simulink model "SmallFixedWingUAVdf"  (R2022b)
settings: Solver=ode4  StartTime=0  StopTime=stoptime  FixedStep=0.001  RelTol=1e-3  EnableMultiTasking=on
PreLoadFcn:
  | asbswarm_vehicledata; % load in workspace variables
PostLoadFcn:
  | open_system([gcs,'/MATLAB Animation Display/MATLAB',10,'Animation']);
InitFcn:
  | InitDatactrl
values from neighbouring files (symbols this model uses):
  env = struct    [InitDatactrl.m]
  F = Fattr + Frep    [APF.m]
  q = ix-1    [bspline_deboor.m]
  SenorSampleTime = 0.01    [InitDatactrl.m]
  sensors = struct    [InitDatactrl.m]
  uav = struct    [InitDatactrl.m]    (also in InitDatactrldf.m)
undefined symbols (not defined in the file or in its folder): Busy, Continuous, DiscIntNeverNeededParam, Dryden, Earth, Light, MIL, Newton, pa28, r, Raphson, sigbuilder_block, Wait, WGS84
libraries: simulink x37, aerolibactuator x10, sharedtransform x6, aerolibatmos2 x4, aerolibasang x4, aerolibwind2 x4, aerolibtransform2 x3, aerolibconvert2 x3, aerolibfltsims x2, shared6dof x2, aerolibnav x2, aerolibanimutils x1
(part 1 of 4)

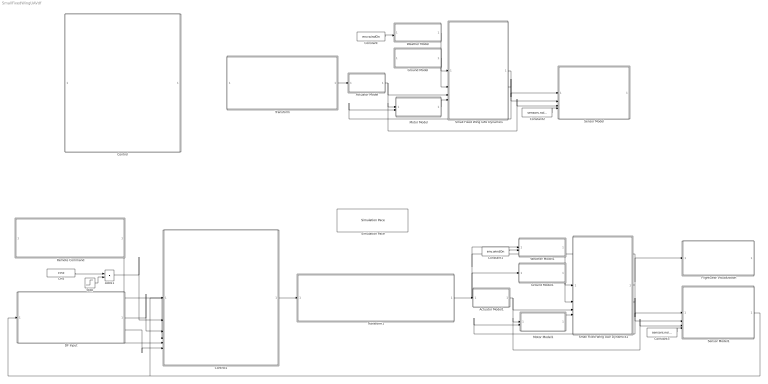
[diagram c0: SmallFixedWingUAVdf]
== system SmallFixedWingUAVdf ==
  Actuator Model : Subsystem  Commented=on
  Actuator Model1 : Subsystem
  Add11 : Sum
  CH5 : Constant  Value=1550  OutDataTypeStr=single
  Constant : Constant  Commented=on  Value=env.windOn
  Constant1 : Constant  Value=env.windOn
  Constant2 : Constant  Commented=on  Value=sensors.noiseOn
  Constant3 : Constant  Value=sensors.noiseOn
  Control : Subsystem  Commented=on
  Control1 : Subsystem
  DF Input : Subsystem
  FlightGear Visualization : Subsystem
  Ground Model : Subsystem  Commented=on
  Ground Model1 : Subsystem
  Motor Model : Subsystem  Commented=on
  Motor Model1 : Subsystem
  Remote Command : Subsystem
  Sensor Model : Subsystem  Commented=on
  Sensor Model1 : Subsystem
  Simulation Pace : aerolibanimutils/Simulation Pace  SimulationPace=1  SleepMode=Busy-Wait  OutputPaceError=off  SampleTime=-1
  Small Fixed Wing UAV Dynamics : Subsystem  Commented=on
  Small Fixed Wing UAV Dynamics1 : Subsystem
  Step : Step  Time=0  After=-100  SampleTime=0
  Transform : Subsystem  Commented=on
  Transform1 : Subsystem
  Weather Model : Subsystem  Commented=on
  Weather Model1 : Subsystem
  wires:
  Small Fixed Wing UAV Dynamics/1(UAVState) -> Sensor Model/1(UAVState)
  Step/1 -> Add11/2
  Motor Model/1(Motor F_M) -> Small Fixed Wing UAV Dynamics/4(Motor Thrust)
  Small Fixed Wing UAV Dynamics/2(AirData) -> Motor Model/2(Air Data), Sensor Model/2(AirData)
  Transform/1(Actuator_act) -> Actuator Model/1(CtrlCmds)
  Actuator Model/1(CtrlSurfaces) -> Small Fixed Wing UAV Dynamics/3(CtrlSurfaces), Sensor Model/3(CtrlSurfaces), Motor Model/1(Ctrl Surfaces)
  Constant2/1 -> Sensor Model/4(if Noise)
  Weather Model/1(Wind_e) -> Small Fixed Wing UAV Dynamics/1(Wind_e)
  Constant/1 -> Weather Model/2(if Wind On)
  CH5/1 -> Add11/1
  Ground Model/1(if Ground) -> Small Fixed Wing UAV Dynamics/2(Ground Detection)
  Actuator Model1/1(CtrlSurfaces) -> Small Fixed Wing UAV Dynamics1/3(CtrlSurfaces), Sensor Model1/3(CtrlSurfaces), Motor Model1/1(Ctrl Surfaces)
  Transform1/1(Actuator_act) -> Actuator Model1/1(CtrlCmds)
  Small Fixed Wing UAV Dynamics1/2(AirData) -> Motor Model1/2(Air Data), Sensor Model1/2(AirData)
  Control1/1(Actuator) -> Transform1/1(Actuator_cmd)
  Constant3/1 -> Sensor Model1/4(if Noise)
  Motor Model1/1(Motor F_M) -> Small Fixed Wing UAV Dynamics1/4(Motor Thrust)
  Ground Model1/1(if Ground) -> Small Fixed Wing UAV Dynamics1/2(Ground Detection)
  Constant1/1 -> Weather Model1/2(if Wind On)
  Weather Model1/1(Wind_e) -> Small Fixed Wing UAV Dynamics1/1(Wind_e)
  Small Fixed Wing UAV Dynamics1/1(UAVState) -> FlightGear Visualization/1(UAVState), Weather Model1/1(UavState), Ground Model1/1(UavState), Sensor Model1/1(UAVState)
  Remote Command/1(Command) -> Control1/1(Command)
  Add11/1 -> Control1/2(ch_switch)
  DF Input/1(RollCmd_Nav) -> Control1/3(RollCmd)
  DF Input/2(AltitudeCmd_Nav) -> Control1/5(AltitudeCmd)
  DF Input/3(AccCmd_Nav) -> Control1/7(AccCmd)
  Sensor Model1/1(SensorData) -> DF Input/1(SensorData), Control1/4(SensorData)

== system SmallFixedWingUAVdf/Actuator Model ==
  note: Simple Actuator Model
  CtrlCmds : Inport
  Bus Creator1 : BusCreator  Inputs=5
  Bus Selector : BusSelector  OutputSignals=elevatorCmd,aileronCmd,rudderCmd,flapCmd,throttleCmd
  Data Type Conversion{1..4,7} (5 alike) : DataTypeConversion  OutDataTypeStr=double
  Linear Second Order Actuators : aerolibactuator/Linear Second-Order Actuator  wn_fin=35  z_fin=0.75  fin_act_0=0  fin_act_vel=0
  Linear Second-Order Actuator{1..4} (4 alike) : aerolibactuator/Linear Second-Order Actuator  wn_fin=35  z_fin=0.75  fin_act_0=0  fin_act_vel=0
  Signal Specification{,1..3} (4 alike) : SignalSpecification  Unit=rad
  Signal Specification4 : SignalSpecification  Unit=%
  CtrlSurfaces : Outport  VectorParamsAs1DForOutWhenUnconnected=off
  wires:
  CtrlCmds/1 -> Bus Selector/1
  Data Type Conversion7/1 -> Linear Second-Order Actuator4/1
  Data Type Conversion1/1 -> Linear Second-Order Actuator3/1
  Data Type Conversion2/1 -> Linear Second-Order Actuator2/1
  Data Type Conversion3/1 -> Linear Second-Order Actuator1/1
  Data Type Conversion4/1 -> Linear Second Order Actuators/1
  Bus Creator1/1 -> CtrlSurfaces/1
  Bus Selector/1 -> Data Type Conversion7/1  "<elevatorCmd>"
  Linear Second-Order Actuator2/1 -> Signal Specification2/1
  Linear Second-Order Actuator3/1 -> Signal Specification1/1
  Linear Second-Order Actuator1/1 -> Signal Specification3/1
  Linear Second-Order Actuator4/1 -> Signal Specification/1
  Bus Selector/4 -> Data Type Conversion3/1  "<flapCmd>"
  Bus Selector/5 -> Data Type Conversion4/1  "<throttleCmd>"
  Bus Selector/3 -> Data Type Conversion2/1  "<rudderCmd>"
  Bus Selector/2 -> Data Type Conversion1/1  "<aileronCmd>"
  Linear Second Order Actuators/1 -> Signal Specification4/1
  Signal Specification/1 -> Bus Creator1/1  "dE"
  Signal Specification1/1 -> Bus Creator1/2  "dA"
  Signal Specification2/1 -> Bus Creator1/3  "dR"
  Signal Specification3/1 -> Bus Creator1/4  "dF"
  Signal Specification4/1 -> Bus Creator1/5  "dT"

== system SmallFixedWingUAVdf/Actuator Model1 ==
  note: Simple Actuator Model
  CtrlCmds : Inport
  Bus Creator1 : BusCreator  Inputs=5
  Bus Selector : BusSelector  OutputSignals=elevatorCmd,aileronCmd,rudderCmd,flapCmd,throttleCmd
  Data Type Conversion{1..4,7} (5 alike) : DataTypeConversion  OutDataTypeStr=double
  Linear Second Order Actuators : aerolibactuator/Linear Second-Order Actuator  wn_fin=35  z_fin=0.75  fin_act_0=0  fin_act_vel=0
  Linear Second-Order Actuator{1..4} (4 alike) : aerolibactuator/Linear Second-Order Actuator  wn_fin=35  z_fin=0.75  fin_act_0=0  fin_act_vel=0
  Signal Specification{,1..3} (4 alike) : SignalSpecification  Unit=rad
  Signal Specification4 : SignalSpecification  Unit=%
  CtrlSurfaces : Outport  VectorParamsAs1DForOutWhenUnconnected=off
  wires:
  CtrlCmds/1 -> Bus Selector/1
  Data Type Conversion7/1 -> Linear Second-Order Actuator4/1
  Data Type Conversion1/1 -> Linear Second-Order Actuator3/1
  Data Type Conversion2/1 -> Linear Second-Order Actuator2/1
  Data Type Conversion3/1 -> Linear Second-Order Actuator1/1
  Data Type Conversion4/1 -> Linear Second Order Actuators/1
  Bus Creator1/1 -> CtrlSurfaces/1
  Bus Selector/1 -> Data Type Conversion7/1  "<elevatorCmd>"
  Linear Second-Order Actuator2/1 -> Signal Specification2/1
  Linear Second-Order Actuator3/1 -> Signal Specification1/1
  Linear Second-Order Actuator1/1 -> Signal Specification3/1
  Linear Second-Order Actuator4/1 -> Signal Specification/1
  Bus Selector/4 -> Data Type Conversion3/1  "<flapCmd>"
  Bus Selector/5 -> Data Type Conversion4/1  "<throttleCmd>"
  Bus Selector/3 -> Data Type Conversion2/1  "<rudderCmd>"
  Bus Selector/2 -> Data Type Conversion1/1  "<aileronCmd>"
  Linear Second Order Actuators/1 -> Signal Specification4/1
  Signal Specification/1 -> Bus Creator1/1  "dE"
  Signal Specification1/1 -> Bus Creator1/2  "dA"
  Signal Specification2/1 -> Bus Creator1/3  "dR"
  Signal Specification3/1 -> Bus Creator1/4  "dF"
  Signal Specification4/1 -> Bus Creator1/5  "dT"

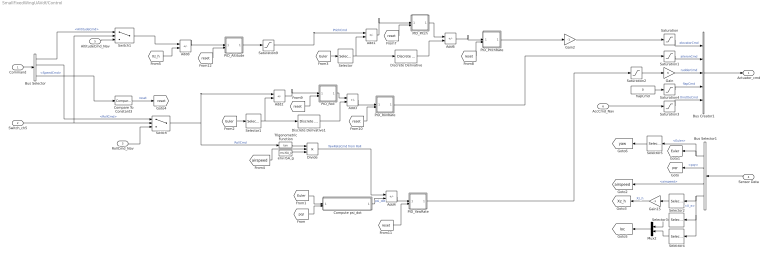
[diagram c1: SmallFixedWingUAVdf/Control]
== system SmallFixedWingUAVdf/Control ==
  Command : Inport
  Switch_ch5 : Inport  Port=2
  RollCmd_Nav : Inport  Port=3
  Sensor Data : Inport  Port=4
  AltitudeCmd_Nav : Inport  Port=5
  AccCmd_Nav : Inport  Port=6
  Add{1..4,6,8} (6 alike) : Sum  Inputs=+-
  Bus Creator1 : BusCreator  Inputs=5
  Bus Selector : BusSelector  OutputSignals=AlititudeCmd,RollCmd,YawRateCmd,SpeedCmd
  Bus Selector1 : BusSelector  OutputSignals=Euler,pqr,airspeed,X_e
  Compare To Constant3 : simulink/Logic and Bit Operations/Compare To Constant  relop=<=  const=0.1  OutDataTypeStr=boolean
  Compute psi_dot : Subsystem
  Discrete Derivative : simulink/Discrete/Discrete Derivative  gainval=1.0  ICPrevScaledInput=0.0  OutMin=[]  OutMax=[]  OutDataType=fixdt(1, 16)  OutScaling=2^-10  DoSatur=off
  Discrete Derivative1 : simulink/Discrete/Discrete Derivative  gainval=1.0  ICPrevScaledInput=0.0  OutMin=[]  OutMax=[]  OutDataType=fixdt(1, 16)  OutScaling=2^-10  DoSatur=off
  Divide : Product  Inputs=*/*
  Gain : Gain
  Gain15 : Gain  Gain=-1
  Gain2 : Gain  Gain=-1
  Mux2 : Mux  Inputs=2
  PID_Altitude : Subsystem
  PID_Pitch : Subsystem
  PID_PitchRate : Subsystem
  PID_Roll : Subsystem
  PID_RollRate : Subsystem
  PID_YawRate : Subsystem
  Saturation : Saturate  UpperLimit=uav.elevator.max  LowerLimit=uav.elevator.min
  Saturation1 : Saturate  UpperLimit=uav.aileron.max  LowerLimit=uav.aileron.min
  Saturation2 : Saturate  UpperLimit=uav.rudder.max  LowerLimit=uav.rudder.min
  Saturation3 : Saturate  UpperLimit=uav.throttlepercent.max  LowerLimit=uav.throttlepercent.min
  Saturation4 : Saturate  UpperLimit=uav.flap.max  LowerLimit=uav.flap.min
  Saturation9 : Saturate  UpperLimit=uav.attitudectrlmax.pitch  LowerLimit=-uav.attitudectrlmax.pitch
  Selector : Selector  InputPortWidth=3  IndexOptions=Index vector (dialog)  Indices=2  OutputSizes=1
  Selector1 : Selector  InputPortWidth=3  IndexOptions=Index vector (dialog)  Indices=1  OutputSizes=1
  Selector2 : Selector  InputPortWidth=3  IndexOptions=Index vector (dialog)  Indices=3  OutputSizes=1
  Selector3 : Selector  InputPortWidth=3  IndexOptions=Index vector (dialog)  Indices=1  OutputSizes=1
  Selector4 : Selector  InputPortWidth=3  IndexOptions=Index vector (dialog)  Indices=2  OutputSizes=1
  Selector5 : Selector  InputPortWidth=3  IndexOptions=Index vector (dialog)  Indices=3  OutputSizes=1
  Switch : Switch  Criteria=u2 > Threshold  Threshold=1500
  Switch1 : Switch  Criteria=u2 > Threshold  Threshold=1500
  Trigonometric Function : Trigonometry  Operator=tan
  env.ISA_g : Constant  Value=env.ISA_g
  flapCmd : Constant  Value=0  OutDataTypeStr=double
  Actuator_cmd : Outport
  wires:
  Saturation1/1 -> Bus Creator1/2  "aileronCmd"
  Add1/1 -> PID_Pitch/1(x)
  Selector3/1 -> Mux2/1
  Bus Selector1/4 -> Selector3/1, Selector4/1, Selector2/1  "<X_e>"
  PID_PitchRate/1(y) -> Gain2/1
  Bus Selector1/1 -> Selector5/1, [Euler]  "<Euler>"
  PID_Altitude/1(y) -> Saturation9/1
  RollCmd_Nav/1 -> Switch/3
  Saturation9/1 -> Add1/1  "PtichCmd"
  Add8/1 -> PID_Altitude/1(x)
  Gain15/1 -> [Xz_h]  "Xz_h"
  [pqr] -> Compute psi_dot/2(G)
  Gain/1 -> Bus Creator1/3  "rudderCmd"
  Selector/1 -> Discrete Derivative/1, Add1/2
  [Xz_h] -> Add8/2
  flapCmd/1 -> Saturation4/1
  [reset] -> PID_Pitch/2(reset_i)
  Bus Selector/2 -> Switch/1  "<RollCmd>"
  Compute psi_dot/1(psi_dot) -> Add4/2  "psi_dot"
  Add6/1 -> PID_PitchRate/1(x)
  Selector2/1 -> Gain15/1
  Bus Selector1/2 -> [pqr]  "<pqr>"
  Selector4/1 -> Mux2/2
  [Euler] -> Compute psi_dot/1(Euler)
  Saturation3/1 -> Bus Creator1/5  "throttleCmd"
  [Euler] -> Selector/1
  Sensor Data/1 -> Bus Selector1/1
  env.ISA_g/1 -> Divide/3
  Add4/1 -> PID_YawRate/1(x)
  [airspeed] -> Divide/2
  Switch/1 -> Add2/1, Trigonometric Function/1  "RollCmd"
  Saturation4/1 -> Bus Creator1/4  "flapCmd"
  Saturation/1 -> Bus Creator1/1  "elevatorCmd"
  PID_Pitch/1(y) -> Add6/1
  Saturation2/1 -> Gain/1
  Discrete Derivative/1 -> Add6/2
  Gain2/1 -> Saturation/1
  Bus Selector/4 -> Compare To Constant3/1  "<SpeedCmd>"
  Divide/1 -> Add4/1  "YawRateCmd from Roll"
  [reset] -> PID_Altitude/2(reset_i)
  PID_YawRate/1(y) -> Saturation2/1
  [reset] -> PID_YawRate/2(reset_i)
  [reset] -> PID_PitchRate/2(reset_i)
  Trigonometric Function/1 -> Divide/1
  Bus Selector1/3 -> [airspeed]  "<airspeed>"
  Command/1 -> Bus Selector/1
  Switch_ch5/1 -> Switch/2, Switch1/2
  Bus Creator1/1 -> Actuator_cmd/1
  Compare To Constant3/1 -> [reset]  "reset"
  Mux2/1 -> [loc]
  Selector5/1 -> [yaw]
  Bus Selector/1 -> Switch1/1  "<AlititudeCmd>"
  Switch1/1 -> Add8/1
  AltitudeCmd_Nav/1 -> Switch1/3
  AccCmd_Nav/1 -> Saturation3/1
  Add2/1 -> PID_Roll/1(x)
  Discrete Derivative1/1 -> Add3/2
  [Euler] -> Selector1/1
  [reset] -> PID_Roll/2(reset_i)
  Selector1/1 -> Discrete Derivative1/1, Add2/2
  PID_Roll/1(y) -> Add3/1
  [reset] -> PID_RollRate/2(reset_i)
  Add3/1 -> PID_RollRate/1(x)
  PID_RollRate/1(y) -> Saturation1/1

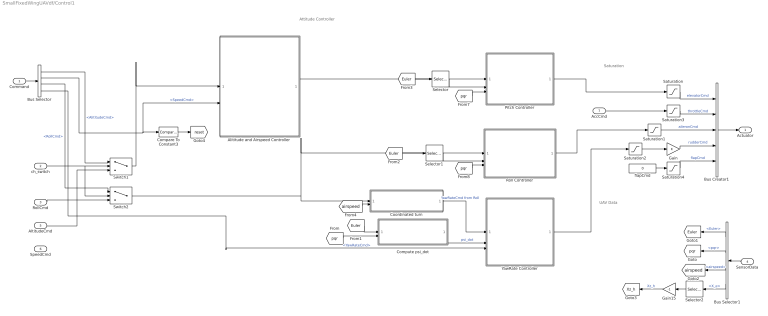
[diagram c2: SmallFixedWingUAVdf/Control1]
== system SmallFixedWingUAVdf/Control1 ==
  note: Attitude Controller
  note: UAV Data
  note: Saturation
  Command : Inport
  ch_switch : Inport  Port=2
  RollCmd : Inport  Port=3
  SensorData : Inport  Port=4
  AltitudeCmd : Inport  Port=5
  SpeedCmd : Inport  Port=6
  AccCmd : Inport  Port=7
  Alititude and Airspeed Controller : Subsystem
  Bus Creator1 : BusCreator  Inputs=5
  Bus Selector : BusSelector  OutputSignals=AlititudeCmd,SpeedCmd,RollCmd,YawRateCmd
  Bus Selector1 : BusSelector  OutputSignals=Euler,pqr,airspeed,X_e
  Compare To Constant3 : simulink/Logic and Bit Operations/Compare To Constant  relop=<=  const=0.2  OutDataTypeStr=boolean
  Compute psi_dot : Subsystem
  Coordinated turn : Subsystem
  Gain : Gain
  Gain15 : Gain  Gain=-1
  Pitch Controller : Subsystem
  Roll Controller : Subsystem
  Saturation : Saturate  UpperLimit=uav.elevator.max  LowerLimit=uav.elevator.min
  Saturation1 : Saturate  UpperLimit=uav.aileron.max  LowerLimit=uav.aileron.min
  Saturation2 : Saturate  UpperLimit=uav.rudder.max  LowerLimit=uav.rudder.min
  Saturation3 : Saturate  UpperLimit=uav.throttlepercent.max  LowerLimit=uav.throttlepercent.min
  Saturation4 : Saturate  UpperLimit=uav.flap.max  LowerLimit=uav.flap.min
  Selector : Selector  InputPortWidth=3  IndexOptions=Index vector (dialog)  Indices=2  OutputSizes=1
  Selector1 : Selector  InputPortWidth=3  IndexOptions=Index vector (dialog)  Indices=1  OutputSizes=1
  Selector2 : Selector  InputPortWidth=3  IndexOptions=Index vector (dialog)  Indices=3  OutputSizes=1
  Switch1 : Switch  Criteria=u2 > Threshold  Threshold=1500
  Switch2 : Switch  Criteria=u2 > Threshold  Threshold=1500
  YawRate Controller : Subsystem
  flapCmd : Constant  Value=0  OutDataTypeStr=double
  Actuator : Outport
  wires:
  Bus Selector1/3 -> [airspeed]  "<airspeed>"
  Pitch Controller/1(elevatorCmd) -> Saturation/1
  [airspeed] -> Coordinated turn/2(<airpseed>)
  [pqr] -> Roll Controller/3(pqr)
  [pqr] -> Pitch Controller/3(pqr)
  Saturation4/1 -> Bus Creator1/5  "flapCmd"
  [Euler] -> Compute psi_dot/1(Euler)
  Bus Selector/1 -> Switch1/1  "<AlititudeCmd>"
  Saturation/1 -> Bus Creator1/1  "elevatorCmd"
  Selector/1 -> Pitch Controller/2(Pitch act)
  Selector1/1 -> Roll Controller/2(Roll act)
  SensorData/1 -> Bus Selector1/1
  Bus Selector1/4 -> Selector2/1  "<X_e>"
  Saturation3/1 -> Bus Creator1/2  "throttleCmd"
  Compare To Constant3/1 -> [reset]
  YawRate Controller/1(rudderCmd) -> Saturation2/1
  Roll Controller/1(aileronCmd) -> Saturation1/1
  Bus Selector1/2 -> [pqr]  "<pqr>"
  [pqr] -> Compute psi_dot/2(G)
  flapCmd/1 -> Saturation4/1
  Selector2/1 -> Gain15/1
  Command/1 -> Bus Selector/1
  Bus Selector/4 -> YawRate Controller/3(<YawRateCmd>)  "<YawRateCmd>"
  [Euler] -> Selector1/1
  Saturation1/1 -> Bus Creator1/3  "aileronCmd"
  Bus Selector1/1 -> [Euler]  "<Euler>"
  Bus Selector/2 -> Alititude and Airspeed Controller/2(<SpeedCmd>), Compare To Constant3/1  "<SpeedCmd>"
  Bus Creator1/1 -> Actuator/1
  Gain/1 -> Bus Creator1/4  "rudderCmd"
  [Euler] -> Selector/1
  Compute psi_dot/1(psi_dot) -> YawRate Controller/2(psi_dot)  "psi_dot"
  Gain15/1 -> [Xz_h]  "Xz_h"
  Coordinated turn/1(YawRateCmd) -> YawRate Controller/1(psi_dot Cmd)  "YawRateCmd from Roll"
  Bus Selector/3 -> Switch2/1  "<RollCmd>"
  Saturation2/1 -> Gain/1
  Alititude and Airspeed Controller/1(pitchout) -> Pitch Controller/1(Pitch cmd)
  ch_switch/1 -> Switch2/2, Switch1/2
  AltitudeCmd/1 -> Switch1/3
  RollCmd/1 -> Switch2/3
  Switch1/1 -> Alititude and Airspeed Controller/1(<AlititudeCmd>)
  AccCmd/1 -> Saturation3/1
  Switch2/1 -> Coordinated turn/1(<RollCmd>), Roll Controller/1(Roll cmd)

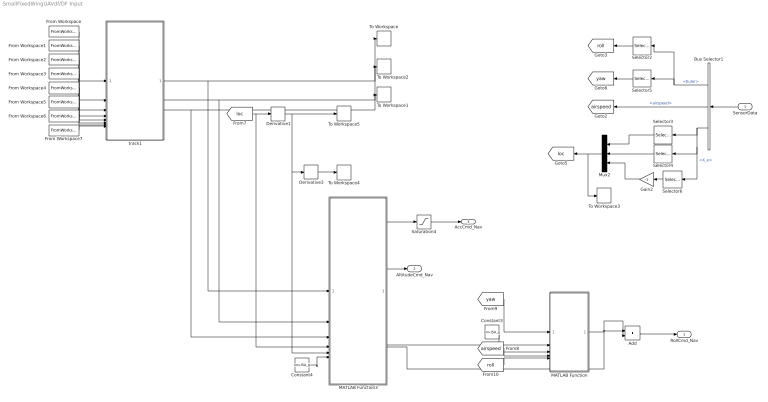
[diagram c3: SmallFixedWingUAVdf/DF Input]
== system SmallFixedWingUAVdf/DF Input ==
  SensorData : Inport
  Add : Sum
  Bus Selector1 : BusSelector  OutputSignals=Euler,airspeed,X_e
  Constant3 : Constant  Value=env.ISA_g
  Constant4 : Constant  Value=env.ISA_g
  Derivative1 : Derivative
  Derivative3 : Derivative
  From Workspace : FromWorkspace  VariableName=xts  SampleTime=-1
  From Workspace1 : FromWorkspace  VariableName=yts  SampleTime=-1
  From Workspace2 : FromWorkspace  VariableName=dxts  SampleTime=-1
  From Workspace3 : FromWorkspace  VariableName=dyts  SampleTime=-1
  From Workspace4 : FromWorkspace  VariableName=ddxts  SampleTime=-1
  From Workspace5 : FromWorkspace  VariableName=ddyts  SampleTime=-1
  From Workspace6 : FromWorkspace  VariableName=dddxts  SampleTime=-1
  From Workspace7 : FromWorkspace  VariableName=dddyts  SampleTime=-1
  Gain2 : Gain  Gain=-1
  MATLAB Function : MATLAB Function  TreatAsAtomicUnit=on
  MATLAB Function3 : MATLAB Function  TreatAsAtomicUnit=on
  Mux2 : Mux  Inputs=3
  Saturation4 : Saturate  UpperLimit=30  LowerLimit=-30
  Selector2 : Selector  InputPortWidth=3  IndexOptions=Index vector (dialog)  Indices=1  OutputSizes=1
  Selector3 : Selector  InputPortWidth=3  IndexOptions=Index vector (dialog)  Indices=1  OutputSizes=1
  Selector4 : Selector  InputPortWidth=3  IndexOptions=Index vector (dialog)  Indices=2  OutputSizes=1
  Selector5 : Selector  InputPortWidth=3  IndexOptions=Index vector (dialog)  Indices=3  OutputSizes=1
  Selector6 : Selector  InputPortWidth=3  IndexOptions=Index vector (dialog)  Indices=3  OutputSizes=1
  To Workspace : ToWorkspace  VariableName=Xd  SampleTime=0.1
  To Workspace1 : ToWorkspace  VariableName=Ad  SampleTime=0.1
  To Workspace2 : ToWorkspace  VariableName=Vd  SampleTime=0.1
  To Workspace3 : ToWorkspace  VariableName=X  SampleTime=0.1
  To Workspace4 : ToWorkspace  VariableName=A  SampleTime=0.1
  To Workspace5 : ToWorkspace  VariableName=V  SampleTime=0.1
  track1 : MATLAB Function  TreatAsAtomicUnit=on
  RollCmd_Nav : Outport
  AltitudeCmd_Nav : Outport  Port=2
  AccCmd_Nav : Outport  Port=3
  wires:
  Bus Selector1/3 -> Selector6/1, Selector4/1, Selector3/1  "<X_e>"
  Selector4/1 -> Mux2/2
  Mux2/1 -> [loc], To Workspace3/1
  Bus Selector1/2 -> [airspeed]  "<airspeed>"
  Selector3/1 -> Mux2/1
  Bus Selector1/1 -> Selector2/1, Selector5/1  "<Euler>"
  Selector5/1 -> [yaw]
  SensorData/1 -> Bus Selector1/1
  From Workspace3/1 -> track1/4(dy)
  From Workspace6/1 -> track1/7(dddx)
  From Workspace7/1 -> track1/8(dddy)
  From Workspace1/1 -> track1/2(y)
  track1/2(Vd) -> MATLAB Function3/2(dxd), To Workspace2/1
  From Workspace2/1 -> track1/3(dx)
  track1/1(Xd) -> MATLAB Function3/1(xd), To Workspace/1
  Derivative3/1 -> To Workspace4/1
  From Workspace5/1 -> track1/6(ddy)
  From Workspace4/1 -> track1/5(ddx)
  track1/3(Ad) -> MATLAB Function3/3(ddxd), To Workspace1/1
  From Workspace/1 -> track1/1(x)
  Selector2/1 -> [roll]
  [loc] -> MATLAB Function3/4(x), Derivative1/1
  Selector6/1 -> Gain2/1
  Gain2/1 -> Mux2/3
  Derivative1/1 -> MATLAB Function3/5(dx), Derivative3/1, To Workspace5/1
  MATLAB Function3/2(Hz) -> AltitudeCmd_Nav/1
  Constant4/1 -> MATLAB Function3/6(g)
  Constant3/1 -> MATLAB Function/3(g)
  [airspeed] -> MATLAB Function/4(V)
  MATLAB Function3/1(av1) -> Saturation4/1
  Saturation4/1 -> AccCmd_Nav/1
  [roll] -> MATLAB Function/5(rolldes)
  MATLAB Function/1(roll) -> Add/1
  MATLAB Function3/4(roll) -> Add/2
  Add/1 -> RollCmd_Nav/1
  MATLAB Function3/3(yaw) -> MATLAB Function/2(yawdes)
  [yaw] -> MATLAB Function/1(yaw)

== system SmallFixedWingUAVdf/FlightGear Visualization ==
  UAVState : Inport
  Bus Creator : BusCreator  Commented=on  Inputs=4
  Bus Selector1 : BusSelector  Commented=on  OutputSignals=gps_Lon,gps_Lat,gps_h,Euler
  Bus Selector3 : BusSelector  OutputSignals=Xe,Euler
  Demux : Demux  Commented=on  Outputs=2
  Demux1 : Demux  Outputs=3
  Flat Earth to LLA : aerolibtransform2/Flat Earth to LLA  Commented=on  units=Metric (MKS)  ptype=Earth (WGS84)  F=1/298.257223563  R=6378137  refPosPort=off  LL0=uav.ic.gsLL  psi=0
  FlightGear Preconfigured 6DoF Animation : aerolibfltsims/FlightGear Preconfigured 6DoF Animation  Commented=on  xFlightGearVersion=v2018.1  DestinationIpAddress=127.0.0.1  DestinationPort=5502  SampleTime=-1  packetVersion=24
  Generate Run Script (if FG is installed) : aerolibfltsims/Generate Run Script  Commented=on  Architecture=Default  dataFlow=Send  GeometryModelName=pa28-161  AirportId=KSFO  RunwayId=10L  InitialAltitude=7224  InitialHeading=113  OffsetDistance=4.72  OffsetAzimuth=0  InstallScenery=on  DisableShaders=on  OriginAddress=127.0.0.1  DestinationPort=5502  OriginPort=5505  LocalAddress=127.0.0.1  OutputFileName=runfg.bat  FlightGearBaseDirectory=C:\Program Files\FlightGear
  Mux1 : Mux  Commented=on
  Terminator : Terminator
  To Workspace : ToWorkspace  VariableName=Fly_x  SampleTime=-1
  To Workspace1 : ToWorkspace  VariableName=Fly_y  SampleTime=-1
  XY Graph : Record  FileSettingsInternal="{\"entries\":[{\"content\":{\"excelSettings\":{\"content\":{},\"type\":\"Streamout.ExcelSettings\"}},\"type\":\"Streamout.FileSettingStorage\",\"uuid\":\"072745bd-254a-47ce-a543-42a2ef1763d8\"}],\"packageUris\":[\"http://schema.mathworks.com/mf0/streamout_blocks/R2020a\"],\"version\":\"1.0\"}"  Layout=[1 1]  SignalsInternal="{\"entries\":[{\"content\":{\"signals\":[{\"content\":{\"blockPath\":[\"SmallFixedWingUAVdf/FlightGear Visualization/XY Graph\"],\"channel\":[],\"dimensions\":[1],\"domain\":\"SmallFixedWingUAVdf/FlightGear Visualization/XY Graph\",\"lineColor\":\"#77ac30\",\"plots\":[],\"port\":1,\"sid\":[\"\"],\"signalID\":745,\"signalName\":\"Demux1:1\"},\"type\":\"RecordBlkView.Signal\",\"uuid\":\"ee7632ca-8912-4ea0-b380-ec3a68b88f7d\"},{\"content\":{\"block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"  VisualizationBindings="{\"xyplotplugin\":{\"info\":[{\"series\":[],\"subplotID\":1}]}}"  CompatibilityTag=XY  st=0.1
  Zero level trust : Constant  Value=0
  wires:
  Bus Selector1/3 -> Mux1/3  "<gps_h>"
  Bus Selector1/1 -> Mux1/1  "<gps_Lon>"
  Flat Earth to LLA/1 -> Demux/1  "gps_latLon"
  Zero level trust/1 -> Flat Earth to LLA/2
  Bus Selector1/2 -> Mux1/2  "<gps_Lat>"
  Mux1/1 -> FlightGear Preconfigured 6DoF Animation/1
  Bus Selector1/4 -> Mux1/4  "<Euler>"
  Bus Creator/1 -> Bus Selector1/1
  Bus Selector3/2 -> Bus Creator/4  "<Euler>"
  Demux/1 -> Bus Creator/1  "gps_Lat"
  Demux/2 -> Bus Creator/2  "gps_Lon"
  Flat Earth to LLA/2 -> Bus Creator/3  "gps_h"
  UAVState/1 -> Bus Selector3/1
  Demux1/3 -> Terminator/1
  Demux1/2 -> To Workspace1/1, XY Graph/2
  Bus Selector3/1 -> Demux1/1, Flat Earth to LLA/1  "<Xe>"
  Demux1/1 -> To Workspace/1, XY Graph/1

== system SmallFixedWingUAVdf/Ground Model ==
  UavState : Inport
  Bus Selector1 : BusSelector  OutputSignals=Xe
  Height : Selector  IndexMode=Zero-based  InputPortWidth=3  IndexOptions=Index vector (dialog)  Indices=2  OutputSizes=1
  Simple Ground Detection : MATLAB Function  TreatAsAtomicUnit=on
  if Ground : Outport  VectorParamsAs1DForOutWhenUnconnected=off
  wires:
  Bus Selector1/1 -> Height/1  "<Xe>"
  UavState/1 -> Bus Selector1/1
  Simple Ground Detection/1(ifGround) -> if Ground/1
  Height/1 -> Simple Ground Detection/1(Xe3)

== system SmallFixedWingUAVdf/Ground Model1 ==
  UavState : Inport
  Bus Selector1 : BusSelector  OutputSignals=Xe
  Height : Selector  IndexMode=Zero-based  InputPortWidth=3  IndexOptions=Index vector (dialog)  Indices=2  OutputSizes=1
  Simple Ground Detection : MATLAB Function  TreatAsAtomicUnit=on
  if Ground : Outport  VectorParamsAs1DForOutWhenUnconnected=off
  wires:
  Bus Selector1/1 -> Height/1  "<Xe>"
  UavState/1 -> Bus Selector1/1
  Simple Ground Detection/1(ifGround) -> if Ground/1
  Height/1 -> Simple Ground Detection/1(Xe3)

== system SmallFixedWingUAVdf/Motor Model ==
  Ctrl Surfaces : Inport
  Air Data : Inport  Port=2
  Bus Selector : BusSelector  OutputSignals=dT
  Bus Selector1 : BusSelector  OutputSignals=airpseed
  Constant : Constant  Value=[0 0 0]
  Engine Model : Subsystem
  Mux : Mux  Inputs=2
  Motor F_M : Outport  VectorParamsAs1DForOutWhenUnconnected=off
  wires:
  Bus Selector1/1 -> Engine Model/2(Airspeed)  "<airpseed>"
  Ctrl Surfaces/1 -> Bus Selector/1
  Engine Model/1(Thrust_b) -> Mux/1
  Constant/1 -> Mux/2
  Air Data/1 -> Bus Selector1/1
  Bus Selector/1 -> Engine Model/1(dt)  "<dT>"
  Mux/1 -> Motor F_M/1

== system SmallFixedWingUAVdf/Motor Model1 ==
  Ctrl Surfaces : Inport
  Air Data : Inport  Port=2
  Bus Selector : BusSelector  OutputSignals=dT
  Bus Selector1 : BusSelector  OutputSignals=airpseed
  Constant : Constant  Value=[0 0 0]
  Mux : Mux  Inputs=2
  Prop Model : Subsystem
  Motor F_M : Outport  VectorParamsAs1DForOutWhenUnconnected=off
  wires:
  Bus Selector1/1 -> Prop Model/2(Airspeed)  "<airpseed>"
  Ctrl Surfaces/1 -> Bus Selector/1
  Prop Model/1(Thrust_b) -> Mux/1
  Constant/1 -> Mux/2
  Air Data/1 -> Bus Selector1/1
  Bus Selector/1 -> Prop Model/1(dt)  "<dT>"
  Mux/1 -> Motor F_M/1

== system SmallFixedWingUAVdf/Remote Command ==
  Add10 : Sum
  Add5 : Sum
  Add9 : Sum
  AlititudeCH2 : Constant  Value=1500  OutDataTypeStr=single
  Bus Creator3 : BusCreator  Inputs=4
  Conversion{2..5} (4 alike) : DataTypeConversion  OutDataTypeStr=double
  InputConditioning : Subsystem
  RollCH1 : Constant  Value=1500  OutDataTypeStr=single
  Signal Builder : Subsystem  Tag=STV Subsys  LoadFcn=sigbuilder_block('load');  StartFcn=sigbuilder_block('start');  StopFcn=sigbuilder_block('stop');  ClipboardFcn=sigbuilder_block('clipboard');  mask(Sigbuilder block){tuvar=[0:10]}
      mask help: Simulink:masks:SigbuilderBlock_MD
      mask init:
      | if ~strcmp(get_param(bdroot(gcbh),'SimulationStatus'),'stopped') tuvar = sigbuilder_block('maskInit'); end
  Signal Builder1 : Subsystem  Tag=STV Subsys  LoadFcn=sigbuilder_block('load');  StartFcn=sigbuilder_block('start');  StopFcn=sigbuilder_block('stop');  ClipboardFcn=sigbuilder_block('clipboard');  mask(Sigbuilder block){tuvar=[0:10]}
      mask help: Simulink:masks:SigbuilderBlock_MD
      mask init:
      | if ~strcmp(get_param(bdroot(gcbh),'SimulationStatus'),'stopped') tuvar = sigbuilder_block('maskInit'); end
  Signal Builder2 : Subsystem  Tag=STV Subsys  LoadFcn=sigbuilder_block('load');  StartFcn=sigbuilder_block('start');  StopFcn=sigbuilder_block('stop');  ClipboardFcn=sigbuilder_block('clipboard');  mask(Sigbuilder block){tuvar=[0:10]}
      mask help: Simulink:masks:SigbuilderBlock_MD
      mask init:
      | if ~strcmp(get_param(bdroot(gcbh),'SimulationStatus'),'stopped') tuvar = sigbuilder_block('maskInit'); end
  Signal Builder3 : Subsystem  Tag=STV Subsys  LoadFcn=sigbuilder_block('load');  StartFcn=sigbuilder_block('start');  StopFcn=sigbuilder_block('stop');  ClipboardFcn=sigbuilder_block('clipboard');  mask(Sigbuilder block){tuvar=[0:10]}
      mask help: Simulink:masks:SigbuilderBlock_MD
      mask init:
      | if ~strcmp(get_param(bdroot(gcbh),'SimulationStatus'),'stopped') tuvar = sigbuilder_block('maskInit'); end
  SpeedCH3 : Constant  Value=1500  OutDataTypeStr=double
  Sum3 : Sum
  YawRateCH4 : Constant  Value=1500  OutDataTypeStr=single
  Command : Outport
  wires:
  Add5/1 -> Conversion3/1
  Conversion5/1 -> InputConditioning/4(ch4)
  InputConditioning/2(Alititude_d) -> Bus Creator3/1  "AlititudeCmd"
  InputConditioning/3(yawRate_d) -> Bus Creator3/3  "YawRateCmd"
  Bus Creator3/1 -> Command/1
  InputConditioning/1(Roll_d) -> Bus Creator3/2  "RollCmd"
  InputConditioning/4(Speed_d) -> Bus Creator3/4  "SpeedCmd"
  Signal Builder1/1(Signal 1) -> Add5/2
  Add9/1 -> Conversion2/1
  RollCH1/1 -> Add9/1
  Conversion2/1 -> InputConditioning/1("ch1 ")
  Sum3/1 -> Conversion5/1
  AlititudeCH2/1 -> Add5/1
  Add10/1 -> Conversion4/1
  Signal Builder3/1(Signal 1) -> Add9/2
  Conversion3/1 -> InputConditioning/2(ch2)
  Signal Builder/1(Signal 1) -> Add10/2
  Signal Builder2/1(Signal 1) -> Sum3/2
  YawRateCH4/1 -> Sum3/1
  SpeedCH3/1 -> Add10/1
  Conversion4/1 -> InputConditioning/3(ch3)

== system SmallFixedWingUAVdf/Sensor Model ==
  UAVState : Inport
  AirData : Inport  Port=2
  CtrlSurfaces : Inport  Port=3
  if Noise : Inport  Port=4  OutDataTypeStr=double  PortDimensions=1
  "Air Sensor Model " : Subsystem
  Assemble GPS and State Data : Subsystem
  Sensor Noise Model : Subsystem
  SensorData : Outport  VectorParamsAs1DForOutWhenUnconnected=off
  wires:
  CtrlSurfaces/1 -> Assemble GPS and State Data/3(CtrlSurfaces)
  UAVState/1 -> Assemble GPS and State Data/1(UAVState), "Air Sensor Model "/1(uavState)
  Assemble GPS and State Data/1(UAVStateBus) -> Sensor Noise Model/1(UAVState)  "uavState"
  if Noise/1 -> Sensor Noise Model/2(if Noise)
  Sensor Noise Model/1(SensorData) -> SensorData/1
  AirData/1 -> "Air Sensor Model "/2(AirData)
  "Air Sensor Model "/1(AirSensorData) -> Assemble GPS and State Data/2(AirSensorData)

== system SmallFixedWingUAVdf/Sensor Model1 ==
  UAVState : Inport
  AirData : Inport  Port=2
  CtrlSurfaces : Inport  Port=3
  if Noise : Inport  Port=4  OutDataTypeStr=double  PortDimensions=1
  "Air Sensor Model " : Subsystem
  Assemble GPS and State Data : Subsystem
  Sensor Noise Model : Subsystem
  SensorData : Outport  VectorParamsAs1DForOutWhenUnconnected=off
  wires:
  CtrlSurfaces/1 -> Assemble GPS and State Data/3(CtrlSurfaces)
  UAVState/1 -> Assemble GPS and State Data/1(UAVState), "Air Sensor Model "/1(uavState)
  Assemble GPS and State Data/1(UAVStateBus) -> Sensor Noise Model/1(UAVState)  "uavState"
  if Noise/1 -> Sensor Noise Model/2(if Noise)
  Sensor Noise Model/1(SensorData) -> SensorData/1
  AirData/1 -> "Air Sensor Model "/2(AirData)
  "Air Sensor Model "/1(AirSensorData) -> Assemble GPS and State Data/2(AirSensorData)

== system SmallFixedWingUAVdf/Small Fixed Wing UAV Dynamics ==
  Wind_e : Inport
  Ground Detection : Inport  Port=2
  CtrlSurfaces : Inport  Port=3
  Motor Thrust : Inport  Port=4
  6DOF Equations of Motion : Subsystem
  Aerodynamic Forces and Moments : Subsystem
  Sum : Sum  Inputs=++|  SaturateOnIntegerOverflow=on
  UAVState : Outport  VectorParamsAs1DForOutWhenUnconnected=off
  AirData : Outport  Port=2  VectorParamsAs1DForOutWhenUnconnected=off
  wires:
  Motor Thrust/1 -> Sum/1
  Aerodynamic Forces and Moments/1(AirData) -> AirData/1
  Aerodynamic Forces and Moments/2(FM_b) -> Sum/2
  Sum/1 -> 6DOF Equations of Motion/1(FM_b)
  Wind_e/1 -> Aerodynamic Forces and Moments/2(Wind_e)
  CtrlSurfaces/1 -> Aerodynamic Forces and Moments/1(CtrlSurfaces)
  6DOF Equations of Motion/1(UAVState) -> UAVState/1, Aerodynamic Forces and Moments/4(UAVState)
  Ground Detection/1 -> Aerodynamic Forces and Moments/3(Ground Detection)

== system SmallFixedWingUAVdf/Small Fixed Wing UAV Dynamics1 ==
  Wind_e : Inport
  Ground Detection : Inport  Port=2
  CtrlSurfaces : Inport  Port=3
  Motor Thrust : Inport  Port=4
  6DOF Equations of Motion : Subsystem
  Aerodynamic Forces and Moments : Subsystem
  Sum : Sum  Inputs=++|  SaturateOnIntegerOverflow=on
  UAVState : Outport  VectorParamsAs1DForOutWhenUnconnected=off
  AirData : Outport  Port=2  VectorParamsAs1DForOutWhenUnconnected=off
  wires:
  Motor Thrust/1 -> Sum/1
  Aerodynamic Forces and Moments/1(AirData) -> AirData/1
  Aerodynamic Forces and Moments/2(FM_b) -> Sum/2
  Sum/1 -> 6DOF Equations of Motion/1(FM_b)
  Wind_e/1 -> Aerodynamic Forces and Moments/2(Wind_e)
  CtrlSurfaces/1 -> Aerodynamic Forces and Moments/1(CtrlSurfaces)
  6DOF Equations of Motion/1(UAVState) -> UAVState/1, Aerodynamic Forces and Moments/4(UAVState)
  Ground Detection/1 -> Aerodynamic Forces and Moments/3(Ground Detection)

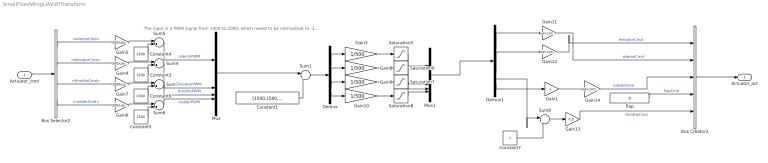
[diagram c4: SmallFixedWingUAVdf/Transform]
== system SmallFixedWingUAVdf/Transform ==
  note: The input is a PWM signal from 1000 to 2000, which needs to be normalized to -1~1.
  Actuator_cmd : Inport
  Bus Creator2 : BusCreator  Inputs=5
  Bus Selector2 : BusSelector  OutputSignals=aileronCmd,elevatorCmd,throttleCmd,rudderCmd
  Constant1 : Constant  Value=[1500,1500,1500,1500]
  Constant3 : Constant  Value=1500
  Constant4 : Constant  Value=1500
  Constant5 : Constant  Value=1500
  Constant6 : Constant  Value=1000
  Constant7 : Constant
  Demux : Demux
  Demux1 : Demux
  Gain1 : Gain  Gain=-1
  Gain{3,8..10} (4 alike) : Gain  Gain=1/500
  Gain11 : Gain  Gain=uav.controlsurfacemax
  Gain12 : Gain  Gain=uav.controlsurfacemax
  Gain13 : Gain  Gain=0.5
  Gain14 : Gain  Gain=uav.controlsurfacemax
  Gain4 : Gain  Gain=500/uav.controlsurfacemax
  Gain5 : Gain  Gain=500/uav.controlsurfacemax
  Gain6 : Gain  Gain=500/uav.controlsurfacemax
  Gain7 : Gain  Gain=1000/uav.throttlepercent.max
  Mux : Mux
  Mux1 : Mux
  Saturation{5..8} (4 alike) : Saturate  UpperLimit=1  LowerLimit=-1
  Sum1 : Sum  Inputs=|+-
  Sum{4..8} (5 alike) : Sum  Inputs=|++
  flap : Constant  Value=0  OutDataTypeStr=double
  Actuator_act : Outport
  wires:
  Sum5/1 -> Mux/1  "aileronPWM"
  Saturation6/1 -> Mux1/2
  Constant1/1 -> Sum1/2
  Bus Selector2/2 -> Gain4/1  "<elevatorCmd>"
  Sum7/1 -> Mux/3  "throttlePWM"
  Constant4/1 -> Sum5/2
  Bus Selector2/1 -> Gain5/1  "<aileronCmd>"
  Constant6/1 -> Sum7/2
  Demux1/1 -> Gain11/1
  Demux1/3 -> Sum8/1
  Saturation5/1 -> Mux1/1
  Gain10/1 -> Saturation8/1
  Mux/1 -> Sum1/1
  Demux/4 -> Gain10/1
  Sum8/1 -> Gain13/1
  Demux/3 -> Gain9/1
  Bus Selector2/3 -> Gain7/1  "<throttleCmd>"
  Demux/1 -> Gain3/1
  Constant3/1 -> Sum4/2
  Gain13/1 -> Bus Creator2/5  "throttleCmd"
  Actuator_cmd/1 -> Bus Selector2/1
  Gain5/1 -> Sum5/1
  Gain11/1 -> Bus Creator2/2  "aileronCmd"
  Gain6/1 -> Sum6/1
  Gain14/1 -> Bus Creator2/3  "rudderCmd"
  Gain12/1 -> Bus Creator2/1  "elevatorCmd"
  Bus Selector2/4 -> Gain6/1  "<rudderCmd>"
  Gain1/1 -> Gain14/1
  Gain8/1 -> Saturation6/1
  Demux1/4 -> Gain1/1
  Constant5/1 -> Sum6/2
  Gain7/1 -> Sum7/1
  flap/1 -> Bus Creator2/4  "flapCmd"
  Demux1/2 -> Gain12/1
  Sum1/1 -> Demux/1
  Constant7/1 -> Sum8/2
  Sum4/1 -> Mux/2  "elevatorPWM"
  Gain4/1 -> Sum4/1
  Sum6/1 -> Mux/4  "rudderPWM"
  Demux/2 -> Gain8/1
  Gain9/1 -> Saturation7/1
  Saturation8/1 -> Mux1/4
  Saturation7/1 -> Mux1/3
  Gain3/1 -> Saturation5/1
  Mux1/1 -> Demux1/1
  Bus Creator2/1 -> Actuator_act/1

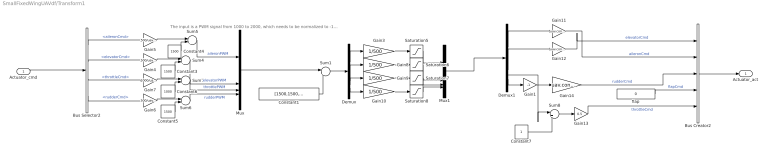
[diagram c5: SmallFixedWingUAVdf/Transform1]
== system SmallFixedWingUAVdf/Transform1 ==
  note: The input is a PWM signal from 1000 to 2000, which needs to be normalized to -1~1.
  Actuator_cmd : Inport
  Bus Creator2 : BusCreator  Inputs=5
  Bus Selector2 : BusSelector  OutputSignals=aileronCmd,elevatorCmd,throttleCmd,rudderCmd
  Constant1 : Constant  Value=[1500,1500,1500,1500]
  Constant3 : Constant  Value=1500
  Constant4 : Constant  Value=1500
  Constant5 : Constant  Value=1500
  Constant6 : Constant  Value=1000
  Constant7 : Constant
  Demux : Demux
  Demux1 : Demux
  Gain1 : Gain  Gain=-1
  Gain{3,8..10} (4 alike) : Gain  Gain=1/500
  Gain11 : Gain  Gain=uav.controlsurfacemax
  Gain12 : Gain  Gain=uav.controlsurfacemax
  Gain13 : Gain  Gain=0.5
  Gain14 : Gain  Gain=uav.controlsurfacemax
  Gain4 : Gain  Gain=500/uav.controlsurfacemax
  Gain5 : Gain  Gain=500/uav.controlsurfacemax
  Gain6 : Gain  Gain=500/uav.controlsurfacemax
  Gain7 : Gain  Gain=1000/uav.throttlepercent.max
  Mux : Mux
  Mux1 : Mux
  Saturation{5..8} (4 alike) : Saturate  UpperLimit=1  LowerLimit=-1
  Sum1 : Sum  Inputs=|+-
  Sum{4..8} (5 alike) : Sum  Inputs=|++
  flap : Constant  Value=0  OutDataTypeStr=double
  Actuator_act : Outport
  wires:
  Mux/1 -> Sum1/1
  Bus Selector2/3 -> Gain7/1  "<throttleCmd>"
  Sum5/1 -> Mux/1  "aileronPWM"
  Constant1/1 -> Sum1/2
  Gain8/1 -> Saturation6/1
  Demux1/4 -> Gain1/1
  Gain5/1 -> Sum5/1
  Actuator_cmd/1 -> Bus Selector2/1
  Constant3/1 -> Sum4/2
  Demux1/1 -> Gain11/1
  Gain3/1 -> Saturation5/1
  Constant6/1 -> Sum7/2
  Bus Selector2/4 -> Gain6/1  "<rudderCmd>"
  Saturation8/1 -> Mux1/4
  Gain7/1 -> Sum7/1
  Sum7/1 -> Mux/3  "throttlePWM"
  Saturation5/1 -> Mux1/1
  Gain6/1 -> Sum6/1
  flap/1 -> Bus Creator2/4  "flapCmd"
  Sum6/1 -> Mux/4  "rudderPWM"
  Gain13/1 -> Bus Creator2/5  "throttleCmd"
  Demux/4 -> Gain10/1
  Demux/2 -> Gain8/1
  Demux/1 -> Gain3/1
  Constant7/1 -> Sum8/2
  Gain9/1 -> Saturation7/1
  Bus Selector2/2 -> Gain4/1  "<elevatorCmd>"
  Sum4/1 -> Mux/2  "elevatorPWM"
  Demux1/2 -> Gain12/1
  Saturation6/1 -> Mux1/2
  Mux1/1 -> Demux1/1
  Gain11/1 -> Bus Creator2/2  "aileronCmd"
  Demux/3 -> Gain9/1
  Sum8/1 -> Gain13/1
  Demux1/3 -> Sum8/1
  Bus Selector2/1 -> Gain5/1  "<aileronCmd>"
  Sum1/1 -> Demux/1
  Constant5/1 -> Sum6/2
  Gain10/1 -> Saturation8/1
  Gain12/1 -> Bus Creator2/1  "elevatorCmd"
  Constant4/1 -> Sum5/2
  Saturation7/1 -> Mux1/3
  Gain14/1 -> Bus Creator2/3  "rudderCmd"
  Gain4/1 -> Sum4/1
  Gain1/1 -> Gain14/1
  Bus Creator2/1 -> Actuator_act/1

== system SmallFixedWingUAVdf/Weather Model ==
  UavState : Inport
  if Wind On : Inport  Port=2
  " Compute Norm" : Subsystem
  Add : Sum  Inputs=2
  Bus Selector3 : BusSelector  OutputSignals=Euler,Xe,Ve
  Constant : Constant  Value=[ 0 0 0]
  Dryden Wind Turbulence Model : aerolibwind2/Dryden Wind Turbulence Model  (Continuous (+q -r))  units=Metric (MKS)  spec=MIL-F-8785C  model=Continuous Dryden (+q -r)  W20=env.windBase/4  Wdeg=env.windDirTurb  TurbProb=10^-2 - Light  L_high=533.4  Wingspan=uav.geometry.span  ts=WindSampleTime  Seed=[23341 23342 23343 23344]  T_on=on
  Gain1 : Gain  Gain=-1
  Get Z1 : Selector  InputPortWidth=3  IndexOptions=Index vector (dialog)  Indices=[3]  OutputSizes=[(-2)]
  "Horizontal Wind Model " : aerolibwind2/Horizontal Wind Model  units=Metric (MKS)  Vw_source=Internal  Vwind=env.windBase  W_source=Internal  Wdeg=env.windDirHor
  RL2B : Subsystem
  Reduce Z Wind : Gain  Gain=[1 1 0.1]
  Rotate to E Frame : Product  Multiplication=Matrix(*)
  Switch : Switch  Criteria=u2 > Threshold  Threshold=0.3
  Terminator : Terminator
  Transpose : Math  Operator=transpose  SignedPower=on
  Wind_e : Outport  Unit=m/s  VectorParamsAs1DForOutWhenUnconnected=off
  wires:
  Bus Selector3/2 -> Get Z1/1  "<Xe>"
  Bus Selector3/1 -> RL2B/1(Euler)  "<Euler>"
  Dryden Wind Turbulence Model/2 -> Terminator/1
  Constant/1 -> Switch/3
  Get Z1/1 -> Gain1/1
  Bus Selector3/3 -> " Compute Norm"/1(<Ve>)  "<Ve>"
  RL2B/1(RL2B) -> Dryden Wind Turbulence Model/3, "Horizontal Wind Model "/1, Transpose/1  "RECEF2B"
  Transpose/1 -> Rotate to E Frame/1
  Rotate to E Frame/1 -> Wind_e/1
  Switch/1 -> Rotate to E Frame/2
  Dryden Wind Turbulence Model/1 -> Reduce Z Wind/1
  " Compute Norm"/1(V) -> Dryden Wind Turbulence Model/2
  UavState/1 -> Bus Selector3/1
  Gain1/1 -> Dryden Wind Turbulence Model/1
  "Horizontal Wind Model "/1 -> Add/2
  Reduce Z Wind/1 -> Add/1
  Add/1 -> Switch/1
  if Wind On/1 -> Switch/2

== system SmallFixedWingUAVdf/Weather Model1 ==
  UavState : Inport
  if Wind On : Inport  Port=2
  " Compute Norm" : Subsystem
  Add : Sum  Inputs=2
  Bus Selector3 : BusSelector  OutputSignals=Euler,Xe,Ve
  Constant : Constant  Value=[ 0 0 0]
  Dryden Wind Turbulence Model : aerolibwind2/Dryden Wind Turbulence Model  (Continuous (+q -r))  units=Metric (MKS)  spec=MIL-F-8785C  model=Continuous Dryden (+q -r)  W20=env.windBase/4  Wdeg=env.windDirTurb  TurbProb=10^-2 - Light  L_high=533.4  Wingspan=uav.geometry.span  ts=WindSampleTime  Seed=[23341 23342 23343 23344]  T_on=on
  Gain1 : Gain  Gain=-1
  Get Z1 : Selector  InputPortWidth=3  IndexOptions=Index vector (dialog)  Indices=[3]  OutputSizes=[(-2)]
  "Horizontal Wind Model " : aerolibwind2/Horizontal Wind Model  units=Metric (MKS)  Vw_source=Internal  Vwind=env.windBase  W_source=Internal  Wdeg=env.windDirHor
  RL2B : Subsystem
  Reduce Z Wind : Gain  Gain=[1 1 0.1]
  Rotate to E Frame : Product  Multiplication=Matrix(*)
  Switch : Switch  Criteria=u2 > Threshold  Threshold=0.3
  Terminator : Terminator
  Transpose : Math  Operator=transpose  SignedPower=on
  Wind_e : Outport  Unit=m/s  VectorParamsAs1DForOutWhenUnconnected=off
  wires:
  Bus Selector3/2 -> Get Z1/1  "<Xe>"
  Bus Selector3/1 -> RL2B/1(Euler)  "<Euler>"
  Dryden Wind Turbulence Model/2 -> Terminator/1
  Constant/1 -> Switch/3
  Get Z1/1 -> Gain1/1
  Bus Selector3/3 -> " Compute Norm"/1(<Ve>)  "<Ve>"
  RL2B/1(RL2B) -> Dryden Wind Turbulence Model/3, "Horizontal Wind Model "/1, Transpose/1  "RECEF2B"
  Transpose/1 -> Rotate to E Frame/1
  Rotate to E Frame/1 -> Wind_e/1
  Switch/1 -> Rotate to E Frame/2
  Dryden Wind Turbulence Model/1 -> Reduce Z Wind/1
  " Compute Norm"/1(V) -> Dryden Wind Turbulence Model/2
  UavState/1 -> Bus Selector3/1
  Gain1/1 -> Dryden Wind Turbulence Model/1
  "Horizontal Wind Model "/1 -> Add/2
  Reduce Z Wind/1 -> Add/1
  Add/1 -> Switch/1
  if Wind On/1 -> Switch/2

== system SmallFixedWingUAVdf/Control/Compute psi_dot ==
  Euler : Inport
  G : Inport  Port=2
  Mux1 : Mux  Inputs=2
  psidot : Fcn  Expr=(u[5]*sin(u[1])+u[6]*cos(u[1]))/cos(u[2])
  psi_dot : Outport  Unit=rad/S  VectorParamsAs1DForOutWhenUnconnected=off
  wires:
  G/1 -> Mux1/2
  psidot/1 -> psi_dot/1  "psi_dot"
  Mux1/1 -> psidot/1
  Euler/1 -> Mux1/1

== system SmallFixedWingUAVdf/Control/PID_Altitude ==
  x : Inport
  reset_i : Inport  Port=2
  Derivative Gain : Gain  DisableCoverage=on  Gain=0  ParamMin=-100  ParamMax=100  OutMin=-100  OutMax=100
  Discrete Derivative : simulink/Discrete/Discrete Derivative  gainval=1.0  ICPrevScaledInput=0.0  OutMin=[]  OutMax=[]  OutDataType=fixdt(1, 16)  OutScaling=2^-10  DoSatur=off
  Discrete-Time Integrator : DiscreteIntegrator  ExternalReset=either  SampleTime=-1  ICPrevOutput=DiscIntNeverNeededParam  ICPrevScaledInput=DiscIntNeverNeededParam
  Gain : Gain  Gain=0.05
  Integral Gain : Gain  DisableCoverage=on  Gain=0
  Sum : Sum  Inputs=+++
  y : Outport  InitialOutput=0  VectorParamsAs1DForOutWhenUnconnected=off
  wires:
  x/1 -> Gain/1, Integral Gain/1, Derivative Gain/1
  Integral Gain/1 -> Discrete-Time Integrator/1
  Derivative Gain/1 -> Discrete Derivative/1
  Gain/1 -> Sum/1
  Sum/1 -> y/1
  Discrete Derivative/1 -> Sum/3
  Discrete-Time Integrator/1 -> Sum/2
  reset_i/1 -> Discrete-Time Integrator/2

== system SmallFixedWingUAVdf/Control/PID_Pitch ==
  x : Inport
  reset_i : Inport  Port=2
  Derivative Gain : Gain  DisableCoverage=on  Gain=0  ParamMin=-100  ParamMax=100  OutMin=-100  OutMax=100
  Discrete Derivative : simulink/Discrete/Discrete Derivative  gainval=1.0  ICPrevScaledInput=0.0  OutMin=[]  OutMax=[]  OutDataType=fixdt(1, 16)  OutScaling=2^-10  DoSatur=off
  Discrete-Time Integrator : DiscreteIntegrator  ExternalReset=either  SampleTime=-1  ICPrevOutput=DiscIntNeverNeededParam  ICPrevScaledInput=DiscIntNeverNeededParam
  Gain : Gain  Gain=3
  Integral Gain : Gain  DisableCoverage=on  Gain=0.1
  Sum : Sum  Inputs=+++
  y : Outport  InitialOutput=0  VectorParamsAs1DForOutWhenUnconnected=off
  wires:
  reset_i/1 -> Discrete-Time Integrator/2
  Discrete-Time Integrator/1 -> Sum/2
  Discrete Derivative/1 -> Sum/3
  Sum/1 -> y/1
  Gain/1 -> Sum/1
  Derivative Gain/1 -> Discrete Derivative/1
  Integral Gain/1 -> Discrete-Time Integrator/1
  x/1 -> Derivative Gain/1, Integral Gain/1, Gain/1

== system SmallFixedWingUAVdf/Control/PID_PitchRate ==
  x : Inport
  reset_i : Inport  Port=2
  Derivative Gain : Gain  DisableCoverage=on  Gain=0.01  ParamMin=-100  ParamMax=100  OutMin=-100  OutMax=100
  Discrete Derivative : simulink/Discrete/Discrete Derivative  gainval=1.0  ICPrevScaledInput=0.0  OutMin=[]  OutMax=[]  OutDataType=fixdt(1, 16)  OutScaling=2^-10  DoSatur=off
  Discrete-Time Integrator : DiscreteIntegrator  ExternalReset=either  SampleTime=-1  LimitOutput=on  UpperSaturationLimit=0.3  LowerSaturationLimit=-0.3  ICPrevOutput=DiscIntNeverNeededParam  ICPrevScaledInput=DiscIntNeverNeededParam
  Gain : Gain  Gain=0.6
  Integral Gain : Gain  DisableCoverage=on  Gain=0.02
  Sum : Sum  Inputs=+++
  y : Outport  InitialOutput=0  VectorParamsAs1DForOutWhenUnconnected=off
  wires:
  x/1 -> Gain/1, Integral Gain/1, Derivative Gain/1
  Integral Gain/1 -> Discrete-Time Integrator/1
  Derivative Gain/1 -> Discrete Derivative/1
  Gain/1 -> Sum/1
  Sum/1 -> y/1
  Discrete Derivative/1 -> Sum/3
  Discrete-Time Integrator/1 -> Sum/2
  reset_i/1 -> Discrete-Time Integrator/2

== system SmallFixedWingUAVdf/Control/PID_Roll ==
  x : Inport
  reset_i : Inport  Port=2
  Derivative Gain : Gain  DisableCoverage=on  Gain=0  ParamMin=-100  ParamMax=100  OutMin=-100  OutMax=100
  Discrete Derivative : simulink/Discrete/Discrete Derivative  gainval=1.0  ICPrevScaledInput=0.0  OutMin=[]  OutMax=[]  OutDataType=fixdt(1, 16)  OutScaling=2^-10  DoSatur=off
  Discrete-Time Integrator : DiscreteIntegrator  ExternalReset=either  SampleTime=-1  ICPrevOutput=DiscIntNeverNeededParam  ICPrevScaledInput=DiscIntNeverNeededParam
  Gain : Gain  Gain=3
  Integral Gain : Gain  DisableCoverage=on  Gain=0.1
  Sum : Sum  Inputs=+++
  y : Outport  InitialOutput=0  VectorParamsAs1DForOutWhenUnconnected=off
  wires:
  x/1 -> Gain/1, Integral Gain/1, Derivative Gain/1
  Integral Gain/1 -> Discrete-Time Integrator/1
  Derivative Gain/1 -> Discrete Derivative/1
  Gain/1 -> Sum/1
  Sum/1 -> y/1
  Discrete Derivative/1 -> Sum/3
  Discrete-Time Integrator/1 -> Sum/2
  reset_i/1 -> Discrete-Time Integrator/2

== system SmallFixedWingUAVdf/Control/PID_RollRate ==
  x : Inport
  reset_i : Inport  Port=2
  Derivative Gain : Gain  DisableCoverage=on  Gain=0.01  ParamMin=-100  ParamMax=100  OutMin=-100  OutMax=100
  Discrete Derivative : simulink/Discrete/Discrete Derivative  gainval=1.0  ICPrevScaledInput=0.0  OutMin=[]  OutMax=[]  OutDataType=fixdt(1, 16)  OutScaling=2^-10  DoSatur=off
  Discrete-Time Integrator : DiscreteIntegrator  ExternalReset=either  SampleTime=-1  LimitOutput=on  UpperSaturationLimit=0.3  LowerSaturationLimit=-0.3  ICPrevOutput=DiscIntNeverNeededParam  ICPrevScaledInput=DiscIntNeverNeededParam
  Gain : Gain  Gain=0.6
  Integral Gain : Gain  DisableCoverage=on  Gain=0.02
  Sum : Sum  Inputs=+++
  y : Outport  InitialOutput=0  VectorParamsAs1DForOutWhenUnconnected=off
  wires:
  reset_i/1 -> Discrete-Time Integrator/2
  Discrete-Time Integrator/1 -> Sum/2
  Discrete Derivative/1 -> Sum/3
  Sum/1 -> y/1
  Gain/1 -> Sum/1
  Derivative Gain/1 -> Discrete Derivative/1
  Integral Gain/1 -> Discrete-Time Integrator/1
  x/1 -> Derivative Gain/1, Integral Gain/1, Gain/1

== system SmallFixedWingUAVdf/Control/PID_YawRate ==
  x : Inport
  reset_i : Inport  Port=2
  Derivative Gain : Gain  DisableCoverage=on  Gain=0  ParamMin=-100  ParamMax=100  OutMin=-100  OutMax=100
  Discrete Derivative : simulink/Discrete/Discrete Derivative  gainval=1.0  ICPrevScaledInput=0.0  OutMin=[]  OutMax=[]  OutDataType=fixdt(1, 16)  OutScaling=2^-10  DoSatur=off
  Discrete-Time Integrator : DiscreteIntegrator  ExternalReset=either  SampleTime=-1  LimitOutput=on  UpperSaturationLimit=0.3  LowerSaturationLimit=-0.3  ICPrevOutput=DiscIntNeverNeededParam  ICPrevScaledInput=DiscIntNeverNeededParam
  Gain : Gain  Gain=0.5
  Integral Gain : Gain  DisableCoverage=on  Gain=0.02
  Sum : Sum  Inputs=+++
  y : Outport  InitialOutput=0  VectorParamsAs1DForOutWhenUnconnected=off
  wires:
  x/1 -> Gain/1, Integral Gain/1, Derivative Gain/1
  Integral Gain/1 -> Discrete-Time Integrator/1
  Derivative Gain/1 -> Discrete Derivative/1
  Gain/1 -> Sum/1
  Sum/1 -> y/1
  Discrete Derivative/1 -> Sum/3
  Discrete-Time Integrator/1 -> Sum/2
  reset_i/1 -> Discrete-Time Integrator/2

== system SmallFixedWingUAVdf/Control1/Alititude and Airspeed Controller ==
  <AlititudeCmd> : Inport
  <SpeedCmd> : Inport  Port=2
  Airspeed Controller : Subsystem
  Saturation9 : Saturate  UpperLimit=uav.attitudectrlmax.pitch  LowerLimit=-uav.attitudectrlmax.pitch
  altitude controller : Subsystem
  pitchout : Outport
  y : Outport  Port=2
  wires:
  <AlititudeCmd>/1 -> altitude controller/1(Alititude cmd)
  [airspeed] -> Airspeed Controller/2(speed act)
  altitude controller/1(pitchout) -> Saturation9/1
  Saturation9/1 -> pitchout/1  "pitchout"
  [Xz_h] -> altitude controller/2(Alititude act)
  Airspeed Controller/1(y) -> y/1
  <SpeedCmd>/1 -> Airspeed Controller/1(Speed cmd)

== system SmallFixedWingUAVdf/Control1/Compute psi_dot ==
  Euler : Inport
  G : Inport  Port=2
  Mux1 : Mux  Inputs=2
  psidot : Fcn  Expr=(u[5]*sin(u[1])+u[6]*cos(u[1]))/cos(u[2])
  psi_dot : Outport  Unit=rad/S  VectorParamsAs1DForOutWhenUnconnected=off
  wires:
  G/1 -> Mux1/2
  psidot/1 -> psi_dot/1  "psi_dot"
  Mux1/1 -> psidot/1
  Euler/1 -> Mux1/1

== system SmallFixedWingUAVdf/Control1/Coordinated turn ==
  <RollCmd> : Inport
  <airpseed> : Inport  Port=2
  Divide : Product  Inputs=*/*
  Trigonometric Function : Trigonometry  Operator=tan
  env.ISA_g : Constant  Value=env.ISA_g
  YawRateCmd : Outport  VectorParamsAs1DForOutWhenUnconnected=off
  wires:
  Trigonometric Function/1 -> Divide/1
  <RollCmd>/1 -> Trigonometric Function/1
  env.ISA_g/1 -> Divide/3
  Divide/1 -> YawRateCmd/1  "YawRateCmd from Roll"
  <airpseed>/1 -> Divide/2
